|Texas Instruments Incorporated
|tmux7349f,  ±60-V Fault-Protected, 8:1 with configurable fault thresholds
[IBIS Ver]   4.1
[File name]   tmux7349f.ibs
[Date]   04/26/22
[File Rev]   1.0
[Source]
| Texas Instruments Incorporated.
| ASC-INT-MPD
| 12500 TI Blvd
| Dallas, TX - 75243
[Notes]   Revision History:
| Rev 1.0: 04/26/22
| - Initial version of the model
| - Model generated from simulations in SPECTRE
| - C_comp although listed in numerical order of value are
|   obtained from varying PVT conditions. For PVT conditions for
|   each specific value refer the buffer description under
|   respective [Model]. IBIS model user is responsible for using
|   appropriate C_comp to simulate for Signal Integrity.
[Disclaimer]
| This model is designed as an aid for customers of Texas Instruments.
| TI and its licensors and suppliers make no warranties, either expressed
| or implied, with respect to this  model, including the warranties of
| merchantability or fitness for a particular purpose. The model is
| provided solely on an "as is" basis. The entire risk as to its quality
| and performance is with the customer.
| This model is subject to change without notice. Texas Instruments
| Incorporated is not responsible for updating this model.
[Copyright]
(C) Copyright 2022 Texas Instruments Incorporated.All rights reserved.
|  Component TMUX7349FPW 20-pin - PW package
|  Part # TMUX7349FPW
[Component]   TMUX7349FPW
[Manufacturer]  TI
[Package]
|   typ   min   max
R_pkg   0.0668   NA   NA
L_pkg   2.1992nH   NA   NA
C_pkg   0.2884pF   NA   NA
[Pin]   signal_name   model_name
   1   A0   inbuf
   2   EN   inbuf
   3   VSS   POWER
   4   S1A   sterm
   5   S2A   sterm
   6   S3A   sterm
   7   S4A   sterm
   8   DA   dterm
   9   VFN   nfault
   10   SF   ofault
   11   FF   ofault
   12   VFP   pfault
   13   DB   dterm
   14   S4B   sterm
   15   S3B   sterm
   16   S2B   sterm
   17   S1B   sterm
   18   VDD   POWER
   19   GND   GND
   20   A1   inbuf
[Series Switch Groups]
On 1 /
On 2 /
On 3 /
On 4 /
Off 1 2 3 4 /
[Series Pin Mapping]  pin_2 model_name function_table_group
 |  4   8   switch_dual_20   1
 |  5   8   switch_dual_20   2
 |  6   8   switch_dual_20   3
 |  7   8   switch_dual_20   4
 | 17   13   switch_dual_20   1
 | 16   13   switch_dual_20   2
 | 15   13   switch_dual_20   3
 | 14   13   switch_dual_20   4
 | 4   8   switch_36   1
 |  5   8   switch_36   2
 |  6   8   switch_36   3
 |  7   8   switch_36   4
 | 17   13   switch_36   1
 | 16   13   switch_36   2
 | 15   13   switch_36   3
 | 14   13   switch_36   4
   4   8   switch_dual_15   1
   5   8   switch_dual_15   2
   6   8   switch_dual_15   3
   7   8   switch_dual_15   4
  17   13   switch_dual_15   1
  16   13   switch_dual_15   2
  15   13   switch_dual_15   3
  14   13   switch_dual_15   4
|   4   8   switch_12   1
 |  5   8   switch_12   2
 |  6   8   switch_12   3
 |  7   8   switch_12   4
 | 17   13   switch_12   1
 | 16   13   switch_12   2
 | 15   13   switch_12   3
 | 14   13   switch_12   4
|  Component TMUX7349FRTJ 20-pin - RTJ package
|  Part # TMUX7349FRTJ
[Component]   TMUX7349FRTJ
[Manufacturer]  TI
[Package]
|   typ   min   max
R_pkg   0.067   NA   NA
L_pkg   0.937nH   NA   NA
C_pkg   0.144pF   NA   NA
[Pin]   signal_name   model_name
   1   VSS   POWER
   2   S1A   sterm
   3   S2A   sterm
   4   S3A   sterm
   5   S4A   sterm
   6   DA   dterm
   7   VFN   nfault
   8   SF   ofault
   9   FF   ofault
   10   VFP   pfault
   11   DB   dterm
   12   S4B   sterm
   13   S3B   sterm
   14   S2B   sterm
   15   S1B   sterm
   16   VDD   POWER
   17   GND   GND
   18   A1   inbuf
   19   A0   inbuf
   20   EN   inbuf
[Series Switch Groups]
On 1 /
On 2 /
On 3 /
On 4 /
Off 1 2 3 4 /
[Series Pin Mapping]  pin_2 model_name function_table_group
|  2   6   switch_dual_20   1
|  3   6   switch_dual_20   2
|  4   6   switch_dual_20   3
|  5   6   switch_dual_20   4
| 15  11   switch_dual_20   1
| 14  11   switch_dual_20   2
| 13  11   switch_dual_20   3
| 12  11   switch_dual_20   4
|   2   6   switch_36   1
|   3   6   switch_36   2
|   4   6   switch_36   3
|   5   6   switch_36   4
|  15  11   switch_36   1
|  14  11   switch_36   2
|  13  11   switch_36   3
|  12  11   switch_36   4
   2   6   switch_dual_15   1
   3   6   switch_dual_15   2
   4   6   switch_dual_15   3
   5   6   switch_dual_15   4
  15  11   switch_dual_15   1
  14  11   switch_dual_15   2
  13  11   switch_dual_15   3
  12  11   switch_dual_15   4
|   2   6   switch_12   1
|   3   6   switch_12   2
|   4   6   switch_12   3
|   5   6   switch_12   4
|  15  11   switch_12   1
|  14  11   switch_12   2
|  13  11   switch_12   3
|  12  11   switch_12   4
[Model Selector] dterm
dterm_dual_20  Use for operation at +/-20V
dterm_36   Use for operation at 36V
dterm_dual_15 Use for operation at +/-15V
dterm_12 Use for operation at 12V
[Model Selector] ofault
ofault_dual_20 Use for operation at +/-20V
ofault_36 Use for operation at 36V
ofault_dual_15 Use for operation at +/-15V
ofault_12 Use for operation at 12V
[Model Selector] sterm
sterm_dual_20 Use for operation at +/-20V
sterm_36 Use for operation at 36V
sterm_dual_15 Use for operation at +/-15V
sterm_12 Use for operation at 12V
[Model Selector] pfault
pfault_dual_20 Use for operation at +/-20V
pfault_36 Use for operation at 36V
pfault_dual_15 Use for operation at +/-15V
pfault_12 Use for operation at 12V
[Model Selector] inbuf
inbuf_dual_20 Use for operation at +/-20V
inbuf_36 Use for operation at 36V
inbuf_dual_15 Use for operation at +/-15V
inbuf_12 Use for operation at 12V
[Model Selector] nfault
nfault_dual_20 Use for operation at +/-20V
| switch_dual_20
[Model]   switch_dual_20
Model_type   Series_switch
|   typ   min   max
C_comp   1.598234e-12   NA   NA
[Voltage Range]   20   NA   NA
[Power Clamp Reference]   20   NA   NA
[Temperature Range]   27   NA   NA
[On]
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[Off]
|   typ   min   max
[R Series]   10G   NA   NA
| switch_36
[Model]   switch_36
Model_type   Series_switch
|   typ   min   max
C_comp   1.598234e-12   NA   NA
[Voltage Range]   36   NA   NA
[Power Clamp Reference]   36   NA   NA
[Temperature Range]   27   NA   NA
[On]
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[Off]
|   typ   min   max
[R Series]   10G   NA   NA
| switch_dual_15
[Model]   switch_dual_15
Model_type   Series_switch
|   typ   min   max
C_comp   1.598234e-12   NA   NA
[Voltage Range]   15   NA   NA
[Power Clamp Reference]   15   NA   NA
[Temperature Range]   27   NA   NA
[On]
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[Off]
|   typ   min   max
[R Series]   10G   NA   NA
| switch_12
[Model]   switch_12
Model_type   Series_switch
|   typ   min   max
C_comp   2.533030e-12   NA   NA
[Voltage Range]   12   NA   NA
[Power Clamp Reference]   12   NA   NA
[Temperature Range]   27   NA   NA
[On]
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[Off]
|   typ   min   max
[R Series]   10G   NA   NA
| Models and submodels in the file (28): ofault_dual_20 (Input), ofault_36 (Input), ofault_dual_15 (Input), ofault_12 (Input), dterm_dual_20 (Terminator), dterm_36 (Terminator), dterm_dual_15 (Terminator), dterm_12 (Terminator), switch_dual_20 (Series_switch), switch_36 (Series_switch), switch_dual_15 (Series_switch), switch_12 (Series_switch), sterm_dual_20 (Terminator), sterm_36 (Terminator), sterm_dual_15 (Terminator), sterm_12 (Terminator), pfault_dual_20 (Input), pfault_36 (Input), pfault_dual_15 (Input), pfault_12 (Input), inbuf_dual_20 (Input), inbuf_36 (Input), inbuf_dual_15 (Input), inbuf_12 (Input), nfault_dual_20 (Input), nfault_36 (Input), nfault_dual_15 (Input), nfault_12 (Input)
